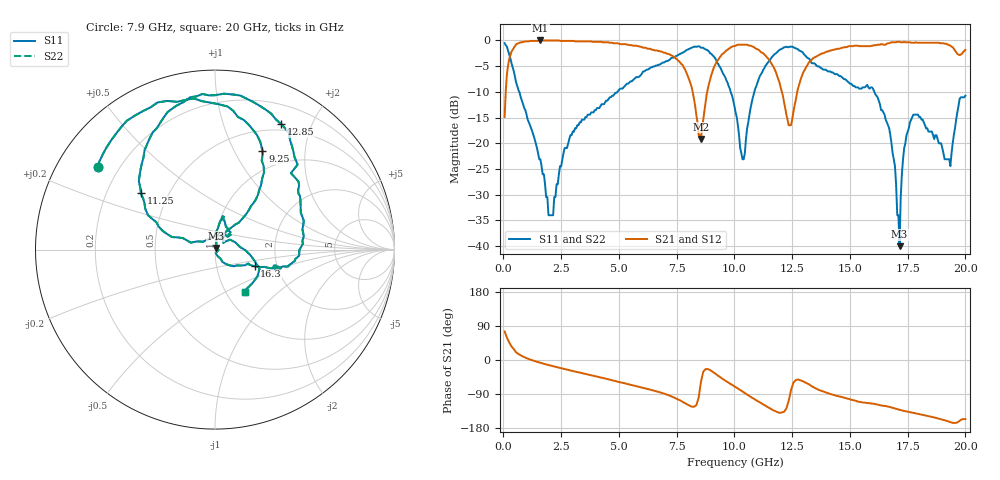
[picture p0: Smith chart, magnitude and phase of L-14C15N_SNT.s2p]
#	mhz	s	ma	r	50
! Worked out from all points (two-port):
!   400 points, 50 MHz to 20 GHz, reference 50 ohm
!   highest |S21| = 0.00 dB at 1.6 GHz (marker M1); lowest = -19.2 dB at 8.55 GHz (marker M2)
!   |S21| within 3 dB of the highest: 290.3 MHz to 7.31 GHz (7.02 GHz wide, 185 % of centre); 13.59 GHz to end of sweep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
!   lowest |S11| = -40.0 dB at 17.15 GHz (marker M3), VSWR 1.02, Z = 50.4 + j0.94 ohm
!   |S11| at or under -10 dB: 684.1 MHz to 4.931 GHz (4.247 GHz wide, 151 % of centre); 9.839 GHz to 10.86 GHz (1.022 GHz wide, 9.87 % of centre); 16.06 GHz to end of sweep
!   |S22| runs from -40.0 to -0.5 dB; largest |S21 - S12| = 0
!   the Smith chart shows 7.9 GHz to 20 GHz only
!   S11 on the Smith chart (normalised r, x): 7.9 GHz: 0.12, +0.31; 9.25 GHz: 0.74, +1.30; 11.25 GHz: 0.35, +0.30; 12.85 GHz: 0.42, +1.58; 16.3 GHz: 1.53, -0.30; 20 GHz: 1.22, -0.63
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50  0.94 169.4  0.18 75.5  0.18 75.5  0.94 169.4
1600  0.07 97.3  1 -7.4  1 -7.4  0.07 97.3
2150  0.02 -149.0  1 -16.4  1 -16.4  0.02 -149.0
3400  0.17 -131.9  0.98 -34.6  0.98 -34.6  0.17 -131.9
6700  0.58 -177.8  0.79 -83.8  0.79 -83.8  0.58 -177.8
6750  0.58 -178.6  0.79 -84.5  0.79 -84.5  0.58 -178.6
6800  0.59 -0.1  0.78 -85.7  0.78 -85.7  0.59 -0.1
6850  0.6 178.5  0.78 -86.8  0.78 -86.8  0.6 178.5
7900  0.8 144.8  0.5 -115.4  0.5 -115.4  0.8 144.8
8550  0.85 104.4  0.11 -57.7  0.11 -57.7  0.85 104.4
9250  0.61 64.3  0.63 -40.1  0.63 -40.1  0.61 64.3
10050  0.2 48.5  0.89 -71.4  0.89 -71.4  0.2 48.5
10400  0.07 126.0  0.91 -85.2  0.91 -85.2  0.07 126.0
11250  0.52 142.7  0.75 -117.2  0.75 -117.2  0.52 142.7
12850  0.79 62.1  0.4 -53.2  0.4 -53.2  0.79 62.1
13350  0.6 45.2  0.65 -69.4  0.65 -69.4  0.6 45.2
16300  0.24 -22.7  0.91 -119.2  0.91 -119.2  0.24 -22.7
16700  0.14 -41.6  0.94 -123.5  0.94 -123.5  0.14 -41.6
17150  0.01 69.0  0.97 -131.6  0.97 -131.6  0.01 69.0
17650  0.17 78.2  0.95 -138.6  0.95 -138.6  0.17 78.2
19350  0.06 39.3  0.89 -163.6  0.89 -163.6  0.06 39.3
20000  0.29 -55.1  0.81 -155.9  0.81 -155.9  0.29 -55.1
